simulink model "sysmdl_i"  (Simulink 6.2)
settings: Solver=ode5  SolverMode=SingleTasking  StartTime=0.0  StopTime=10.0  FixedStep=0.1  RelTol=1e-3  AbsTol=1e-6
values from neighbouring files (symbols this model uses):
  g = 9.8    [ch8_c.m]    (also in ch8_d.m; ch8_h.m; s_xmp2.m)
  k1 = KK(1)    [ch8_d.m]    (also in set_x4a.m = 1; za_podmodel_voz.m = 1; auto_param.m = 7500; auto_param_opt.m = 15000)
  k2 = KK(2)    [ch8_d.m]    (also in set_x4a.m = 2; za_podmodel_voz.m = 2; auto_param.m = 150000; auto_param_opt.m = 150000)
  k3 = KK(3)    [ch8_d.m]    (also in set_x4a.m = 4; za_podmodel_voz.m = 4; INTEG_RK4.M = krm(2)*DERIV(t+0.5*krm(2),y+0.5*k2,par); kovinska_palica_2_RK4.m = 0.5)
  k4 = KK(4)    [ch8_d.m]    (also in INTEG_RK4.M = krm(2)*DERIV(t+krm(2),y+k3,par))
  KI = -KK(5)    [ch8_d.m]
  l = sqrt(dx1^2 + dx2^2)*7.5    [ch8_b.m]    (also in ch8_c.m = 0.5; ch8_d.m = 0.5; ch8_f.m; ch8_h.m = 0.3)
  m = 0.1    [ch8_c.m]    (also in ch8_d.m; ch8_h.m = 0.2; s_xmp3.m = 1; auto_param.m = 500)
  M = 2    [ch8_c.m]    (also in ch8_d.m; s_xmp3.m = 1; Monte_Carlo_PI.m)

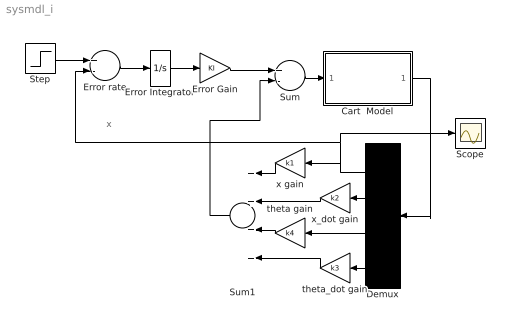
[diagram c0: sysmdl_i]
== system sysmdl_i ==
  note: x
  Cart  Model : Subsystem
  Demux : Demux  Orientation=left
  Error Gain : Gain  Gain=KI
  Error Integrator : Integrator  UpperSaturationLimit=2  LowerSaturationLimit=-2
  Error rate : Sum  Inputs=+-
  Scope : Scope
  Step : Step  SampleTime=0
  Sum : Sum  Inputs=+-
  Sum1 : Sum  Orientation=left  Inputs=++++
  theta gain : Gain  Orientation=left  Gain=k4
  theta_dot gain : Gain  Orientation=left  Gain=k3
  x gain : Gain  Orientation=left  Gain=k1
  x_dot gain : Gain  Orientation=left  Gain=k2
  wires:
  Error rate/1 -> Error Integrator/1
  Cart  Model/1(state  out) -> Demux/1
  Demux/1 -> Scope/1, Error rate/2, x gain/1
  Sum1/1 -> Sum/2
  x gain/1 -> Sum1/1
  x_dot gain/1 -> Sum1/2
  theta gain/1 -> Sum1/3
  theta_dot gain/1 -> Sum1/4
  Demux/4 -> theta_dot gain/1
  Demux/3 -> theta gain/1
  Demux/2 -> x_dot gain/1
  Step/1 -> Error rate/1
  Error Integrator/1 -> Error Gain/1
  Error Gain/1 -> Sum/1
  Sum/1 -> Cart  Model/1(thrust  in)

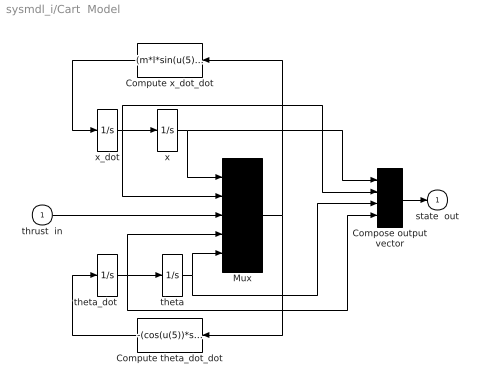
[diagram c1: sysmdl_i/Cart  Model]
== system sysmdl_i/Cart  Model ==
  thrust  in : Inport  Port=1  LatchInput=off
  Compose output vector : Mux
  Compute theta_dot_dot : Fcn  Orientation=left  Expr=-(cos(u(5))*sin(u(5))*m*l*u(4)*u(4)-m*g*sin(u(5))+u(3)*cos(u(5))-g*M*sin(u(5)))/(l*(M+m*sin(u(5))*sin(u(5))))
  Compute x_dot_dot : Fcn  Orientation=left  Expr=(m*l*sin(u(5))*u(4)*u(4)-m*cos(u(5))*g*sin(u(5))+u(3))/(M+m*sin(u(5))*sin(u(5)))
  Mux : Mux  Inputs=5
  theta : Integrator
  theta_dot : Integrator
  x : Integrator
  x_dot : Integrator
  state  out : Outport  InitialOutput=0
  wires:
  thrust  in/1 -> Mux/3
  theta/1 -> Compose output vector/3, Mux/5
  x/1 -> Compose output vector/1, Mux/1
  Compose output vector/1 -> state  out/1
  Mux/1 -> Compute theta_dot_dot/1, Compute x_dot_dot/1
  Compute theta_dot_dot/1 -> theta_dot/1
  Compute x_dot_dot/1 -> x_dot/1
  x_dot/1 -> Compose output vector/2, Mux/2, x/1
  theta_dot/1 -> Compose output vector/4, Mux/4, theta/1
